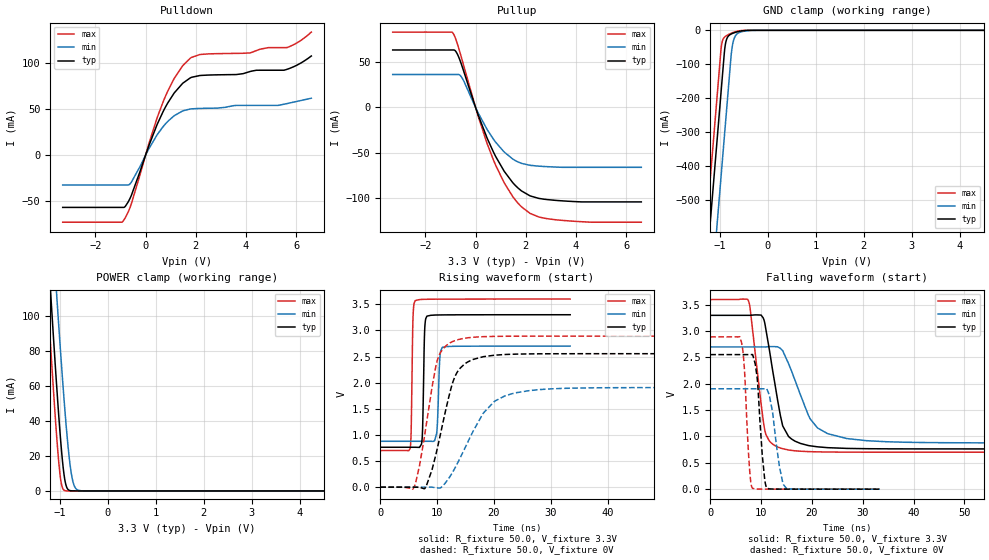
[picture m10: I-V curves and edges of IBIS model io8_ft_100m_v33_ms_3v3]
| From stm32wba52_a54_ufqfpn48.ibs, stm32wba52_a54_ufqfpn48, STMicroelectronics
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[Model]   io8_ft_100m_v33_ms_3v3
Model_type I/O
Polarity   Non-Inverting
Enable   Active-Low
| CAP_THRESHOLD on pad IOFT is "UDTCAPC" :
| Rising=30.0% of vddiom   Falling=70.0% of vddiom
| C_comp min and max val. don't necessarily correlate with the min and max pvt
| but are the smallest and greatest pad capacitance found.
| var   typ   min   max
C_comp   2.72384pF  2.64021pF  2.77561pF
|C_comp_pullup   1.81450pF  1.75560pF  1.84959pF
|C_comp_pulldown   909.34635fF  884.60580fF  926.02020fF
Vinl = 1.35V
Vinh = 1.8V
Vmeas = 1.65V   | Reference voltage for timing measurements
Cref  = 50.0pF   | Timing specification test load capacitance value
Rref  = 1.0MOhm   | Timing specification test load resistance value
Vref  = 1.815V   | Timing specification test load voltage
[Model Spec]
| TIME_THRESHOLD on pin ZIV33M is "CMOS" :
| Rising=50.0% of vddiom   Falling=50.0% of vddiom
Vinl 1.28450V 1.07650V 1.38450V
Vinh 1.79550V 1.49050V 1.94250V
| variable   typ   min   max
[Temperature Range] 25.0 140.0 -40.0
| variable   typ   min   max
[Voltage Range] 3.3V 2.7V 3.6V
| variable   typ   min   max
[POWER Clamp Reference] 3.3V 2.7V 3.6V
| variable   typ   min   max
[GND Clamp Reference] 0V 0V 0V
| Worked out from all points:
|   slope of the pulldown table from 0 to 0.495 V, typ, clamps not added: 14 ohm
|   slope of the pullup table from 0 to 0.495 V, typ, clamps not added: 13.8 ohm
|   GND clamp passes 1 mA (typ) near -0.51 V on its own axis
|   POWER clamp passes 1 mA (typ) near -0.83 V on its own axis
|   rising waveform, R_fixture 50.0, V_fixture 3.3V: 20-80 % time 264ps typ, 347ps min, 237ps max; typ from 0.764 V to 3.3 V
|   falling waveform, R_fixture 50.0, V_fixture 3.3V: 20-80 % time 2.72ns typ, 4.83ns min, 2.13ns max; typ from 3.3 V to 0.764 V
|   rising waveform, R_fixture 50.0, V_fixture 0V: 20-80 % time 3.36ns typ, 5.85ns min, 2.61ns max; typ from 0 V to 2.55 V
|   falling waveform, R_fixture 50.0, V_fixture 0V: 20-80 % time 1.08ns typ, 1.57ns min, 901ps max; typ from 2.55 V to 0 V
[POWER Clamp]
-3.3V     1.123A     1.139A     1.091A
-1.36V    189.2mA    238.8mA    158.1mA
-1.25V    139mA      190.3mA    108.1mA
-1.18V    107.9mA    159.9mA    77.22mA
-1.06V    57.23mA    109.3mA    28.68mA
-980mV    27.6mA     77.28mA    5.935mA
-900mV    6.895mA    47.74mA    242.8uA
-820mV    594.6uA    22.85mA    5.912uA
-760mV    69.41uA    9.714mA    358.6nA
-700mV    7.83uA     2.919mA    21.86nA
-630mV    611.5nA    529.9uA    954.5pA
6.6V      0A         0A         0A
[GND Clamp]
-3.3V     -4.134A    -4.382A    -4.006A
-1.59V    -1.227A    -1.475A    -1.099A
-1.25V    -648.9mA   -896.7mA   -520.9mA
-980mV    -189.9mA   -437.7mA   -61.92mA
-970mV    -172.9mA   -420.7mA   -48.45mA
-910mV    -70.86mA   -318.7mA   -21.03mA
-880mV    -37.23mA   -267.7mA   -17.31mA
-750mV    -9.908mA   -55.25mA   -7.768mA
-710mV    -7.626mA   -27.41mA   -5.608mA
-650mV    -4.885mA   -11.6mA    -3.058mA
-360mV    -31.22uA   -443.6uA   -1.188uA
6.6V      2.31nA     2.655uA    974.6pA
| variable   typ   min   max
[Pullup Reference] 3.3V 2.7V 3.6V
| variable   typ   min   max
[Pulldown Reference] 0V 0V 0V
[Pullup]
-3.3V     63.27mA    36.29mA    82.98mA
-900mV    63.27mA    36.29mA    81.88mA
-750mV    60.02mA    36.29mA    72.1mA
-540mV    45.51mA    32.56mA    52.64mA
120mV     -9.566mA   -6.929mA   -11.25mA
710mV     -49.08mA   -34.92mA   -57.81mA
1.14V     -70.33mA   -49.14mA   -83.06mA
1.48V     -82.86mA   -56.83mA   -98.19mA
1.83V     -91.98mA   -61.62mA   -109.5mA
2.17V     -97.42mA   -63.75mA   -116.7mA
2.85V     -101.5mA   -65.23mA   -122.5mA
6.6V      -104mA     -65.97mA   -126.4mA
[Pulldown]
-3.3V     -56.7mA    -32.4mA    -72.73mA
-890mV    -56.7mA    -32.4mA    -71.32mA
-570mV    -43.94mA   -29.54mA   -52.99mA
120mV     9.474mA    6.407mA    11.48mA
700mV     47.33mA    30.97mA    57.88mA
1.14V     67.41mA    42.74mA    83.2mA
1.78V     83.75mA    50.04mA    105.1mA
2.17V     86.37mA    50.65mA    109.1mA
4.16V     90.65mA    53.91mA    110.8mA
4.9V      92.06mA    53.91mA    116.6mA
5.63V     93.04mA    55.89mA    116.6mA
6.6V      107.5mA    61.71mA    133.4mA
[Ramp]
dV/dt_r 1.53258V/3.33803ns 1.14345V/5.65064ns 1.73412V/2.58801ns
dV/dt_f 1.52157V/2.69175ns 1.09312V/4.66132ns 1.73923V/2.10314ns
R_load = 50.0
| Removed startup time: 0s 0s 0s  .
| Removed end time: 33.4ns.
[Rising Waveform]
R_fixture   = 50.0
V_fixture   = 3.3V
V_fixture_min = 2.7V
V_fixture_max = 3.6V
0s        764mV      878.1mV    701.3mV
5.25ns    764.1mV    878.1mV    742.2mV
5.75ns    764.1mV    878.1mV    3.221V
6.15ns    764.1mV    878.1mV    3.572V
7.35ns    912.9mV    878.1mV    3.594V
7.8ns     2.988V     878.1mV    3.595V
8.2ns     3.273V     878.1mV    3.596V
9.9ns     3.295V     1.02V      3.598V
10.9ns    3.297V     2.675V     3.598V
33.4ns    3.3V       2.7V       3.6V
| Removed startup time: 0s 0s 0s  .
| Removed end time: 188.4ns.
[Falling Waveform]
R_fixture   = 50.0
V_fixture   = 3.3V
V_fixture_min = 2.7V
V_fixture_max = 3.6V
0s        3.3V       2.7V       3.6V
7.45ns    3.3V       2.7V       3.588V
10.4ns    3.253V     2.7V       1.316V
11.55ns   2.69V      2.706V     925.2mV
13.8ns    1.394V     2.672V     781mV
15.4ns    999.8mV    2.383V     743.8mV
19.25ns   829.2mV    1.415V     713.1mV
21.1ns    803.7mV    1.162V     708.1mV
30.75ns   768.1mV    920.5mV    701.7mV
188.4ns   764mV      878.1mV    701.3mV
| Removed startup time: 0s 0s 0s  .
| Removed end time: 98.35ns.
[Rising Waveform]
R_fixture   = 50.0
V_fixture   = 0V
V_fixture_min = 0V
V_fixture_max = 0V
0s        20.88nV    574.1nV    33.14nV
5.75ns    7.995uV    591.5nV    -32.91mV
6.9ns     -2.854mV   924.6nV    409.4mV
8.05ns    9.286mV    7.032uV    1.168V
10.25ns   848mV      -15.75mV   2.497V
12.5ns    1.915V     244.2mV    2.774V
13.8ns    2.243V     506mV      2.827V
20.1ns    2.526V     1.645V     2.886V
26.1ns    2.55V      1.846V     2.89V
98.35ns   2.554V     1.906V     2.89V
| Removed startup time: 0s 0s 0s  .
| Removed end time: 33.35ns.
[Falling Waveform]
R_fixture   = 50.0
V_fixture   = 0V
V_fixture_min = 0V
V_fixture_max = 0V
0s        2.554V     1.906V     2.89V
6.15ns    2.554V     1.906V     2.785V
6.75ns    2.554V     1.906V     2.228V
7.7ns     2.554V     1.906V     417.3mV
8.3ns     2.557V     1.906V     18mV
9.2ns     2.131V     1.906V     2.609mV
10.25ns   626.9mV    1.906V     1.446mV
11.1ns    25.63mV    1.907V     1.106mV
15ns      971.1uV    12.33mV    510.9uV
33.35ns   27.86uV    157.8uV    5.206uV
